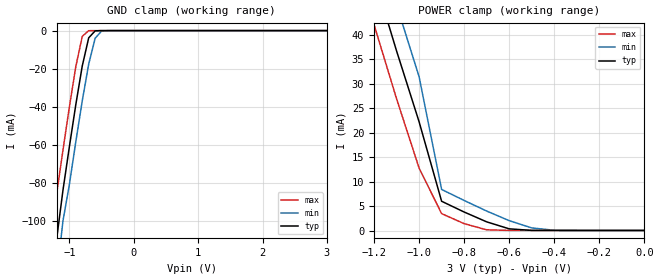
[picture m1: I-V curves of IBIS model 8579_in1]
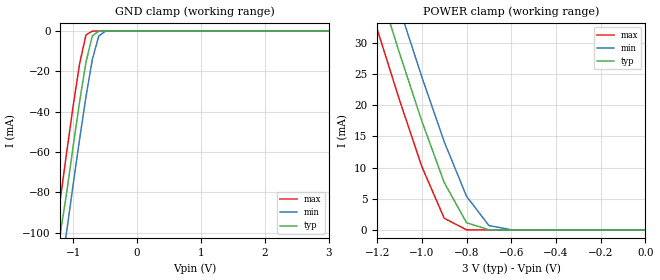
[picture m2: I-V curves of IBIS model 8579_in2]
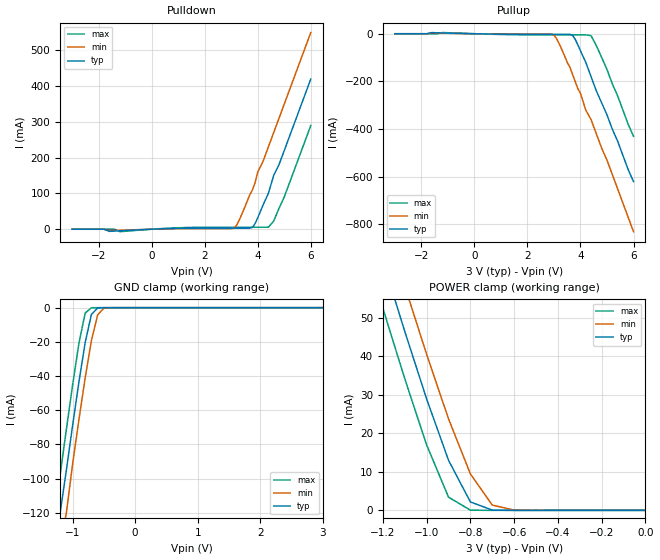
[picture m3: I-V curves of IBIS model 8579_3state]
| IBIS file 4574_3.ibs
[IBIS ver]   3.0
[File name]   4574_3.ibs
[File Rev]   3.0
[Date]   Thursday 7, 2005
[Source]   Hspice simulation by NPC using HA8579 schematics
[Disclaimer]   Data is for modeling purpose only and is not guaranteed.
[Copyright]   SEIKO EPSON Corp.
|   Component RTC-4574SA
[Component]   RTC-4574SA
[Manufacturer]   Seiko Epson Corporation
[Package]
| variable   typ   min   max
R_pkg   3.00m   NA   NA
L_pkg   3.70nH   NA   NA
C_pkg   0.70pF   NA   NA
[Pin]  signal_name   model_name   R_pin   L_pin   C_pin
1   VSS   GND
2   FOUT   8579_3state
|3   NC
|4   NC
|5   NC
|6   NC
7   VDD   POWER
8   CE0   8579_in1
9   AIRQN   8579_od
10   TIRQN   8579_od
11   CLK   8579_in2
12   DATA   8579_io
13   CE1   8579_in2
14   FCON   8579_in2
| Models and submodels in the file (5): 8579_in1 (Input), 8579_in2 (Input), 8579_3state (3-state), 8579_io (I/O), 8579_od (Open_drain)
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|   Model 8579_in1
[Model]   8579_in1
Model_type   Input
Vinl =   0.60V
Vinh =   2.40V
C_comp   8.00pF   8.00pF   8.00pF
[Temperature Range]   25.00   85.00   -40.00
[Voltage Range]   3.00V   2.70V   3.30V
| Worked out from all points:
|   GND clamp passes 1 mA (typ) near -0.62 V on its own axis
|   POWER clamp passes 1 mA (typ) near -0.65 V on its own axis
[GND_clamp]
| voltage   I(typ)   I(min)   I(max)
-3V       -550mA     -570mA     -530mA
-1.3V     -130mA     -150mA     -110mA
-1.2V     -110mA     -130mA     -86.2mA
-1.1V     -83.87mA   -100mA     -62.79mA
-1V       -60.92mA   -80.78mA   -40.05mA
-900mV    -38.82mA   -58.3mA    -18.83mA
-800mV    -18.56mA   -36.84mA   -3.02mA
-700mV    -3.78mA    -17.56mA   -37.75uA
-600mV    -140uA     -3.99mA    -260nA
-500mV    -2.83uA    -250uA     -1.81nA
3V        8.96uA     6.98uA     16.13uA
[POWER_clamp]
| voltage   I(typ)   I(min)   I(max)
-3V       340mA      350mA      340mA
-1.2V     51.94mA    61.35mA    42.1mA
-1.1V     36.73mA    46.14mA    26.95mA
-1V       22.24mA    31.45mA    12.77mA
-900mV    5.98mA     8.4mA      3.45mA
-800mV    3.78mA     6.14mA     1.4mA
-700mV    1.77mA     3.98mA     140uA
-600mV    340uA      2.01mA     17.19uA
-500mV    20.1uA     530uA      16.15uA
-400mV    9.2uA      44.36uA    16.14uA
0V        8.96uA     5.37uA     16.13uA
|   Model 8579_in2
[Model]   8579_in2
Model_type   Input
Vinl =   0.60V
Vinh =   2.40V
C_comp   8.00pF   8.00pF   8.00pF
[Temperature Range]   25.00   85.00   -40.00
[Voltage Range]   3.00V   2.70V   3.30V
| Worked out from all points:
|   GND clamp passes 1 mA (typ) near -0.64 V on its own axis
|   POWER clamp passes 1 mA (typ) near -0.79 V on its own axis
[GND_clamp]
| voltage   I(typ)   I(min)   I(max)
-3V       -540mA     -560mA     -520mA
-1.3V     -130mA     -150mA     -110mA
-1.2V     -100mA     -120mA     -82.91mA
-1.1V     -79.74mA   -98.87mA   -59.57mA
-1V       -56.91mA   -75.91mA   -36.97mA
-900mV    -35.02mA   -53.6mA    -16.13mA
-800mV    -15.33mA   -32.47mA   -1.89mA
-700mV    -2.36mA    -13.97mA   -18.95uA
-600mV    -68.66uA   -2.44mA    -130nA
-500mV    -1.41uA    -130uA     -910pA
3V        3pA        2.02nA     2.7pA
[POWER_clamp]
| voltage   I(typ)   I(min)   I(max)
-3V       260mA      270mA      250mA
-1.2V     39.81mA    47.03mA    32.25mA
-1.1V     28.38mA    35.6mA     20.85mA
-1V       17.46mA    24.55mA    10.16mA
-900mV    7.61mA     14.16mA    1.88mA
-800mV    1.16mA     5.39mA     27.3uA
-700mV    33.67uA    710uA      190nA
-600mV    690nA      33.17uA    1.31nA
0V        3pA        14.76pA    3.3pA
|   Model   8579_3state
[Model]   8579_3state
Model_type   3-state
Polarity   Inverting
C_comp   8.00pF   8.00pF   8.00pF
[Temperature Range]   25   85   -40
[Voltage Range]   3.00V   2.70V   3.30V
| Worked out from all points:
|   slope of the pulldown table from 0 to 0.45 V, typ, clamps not added: 346 ohm
|   slope of the pullup table from 0 to 0.45 V, typ, clamps not added: 474 ohm
|   GND clamp passes 1 mA (typ) near -0.62 V on its own axis
|   POWER clamp passes 1 mA (typ) near -0.74 V on its own axis
[Pulldown]
|   voltage   I(typ)   I(min)   I(max)
-3V       0A         0A         0A
-1.4V     -5.09mA    -3.39mA    0A
-1.2V     -4.49mA    -2.98mA    -6.79mA
3.1V      2.89mA     2.77mA     5.47mA
3.3V      2.9mA      25.15mA    5.48mA
3.8V      5.09mA     110mA      5.49mA
3.9V      15.91mA    130mA      5.49mA
4V        31.8mA     160mA      5.49mA
4.4V      100mA      230mA      5.55mA
4.6V      150mA      270mA      22.48mA
5V        220mA      350mA      90.27mA
6V        420mA      550mA      290mA
[Pullup]
|   voltage   I(typ)   I(min)   I(max)
-3V       0A         0A         0A
-1.2V     3.25mA     2.18mA     5.03mA
3V        -2.47mA    -5.37mA    -4.82mA
3.2V      -2.48mA    -42.34mA   -4.84mA
3.7V      -6.45mA    -170mA     -4.87mA
3.9V      -46.01mA   -230mA     -4.88mA
4V        -71.24mA   -250mA     -4.89mA
4.2V      -120mA     -320mA     -4.9mA
4.4V      -180mA     -360mA     -8.08mA
4.6V      -240mA     -420mA     -50mA
5V        -340mA     -530mA     -150mA
6V        -620mA     -830mA     -430mA
[GND_clamp]
|   voltage   I(typ)   I(min)   I(max)
-3V       -620mA     -650mA     -600mA
-1.3V     -150mA     -170mA     -120mA
-1.2V     -120mA     -140mA     -97.79mA
-1.1V     -94.94mA   -120mA     -71.05mA
-1V       -68.74mA   -91.25mA   -45.09mA
-900mV    -43.52mA   -65.59mA   -20.92mA
-800mV    -20.48mA   -41.13mA   -3.17mA
-700mV    -3.96mA    -19.25mA   -37.79uA
-600mV    -140uA     -4.17mA    -260nA
-500mV    -2.83uA    -250uA     -1.81nA
3V        3.01pA     66.2uA     2.4pA
[POWER_clamp]
|   voltage   I(typ)   I(min)   I(max)
-3V       420mA      430mA      400mA
-1.3V     83.45mA    95.19mA    71.21mA
-1.2V     64.75mA    76.53mA    52.43mA
-1.1V     46.44mA    58.21mA    34.17mA
-1V       28.9mA     40.47mA    16.98mA
-900mV    13mA       23.75mA    3.42mA
-800mV    2.18mA     9.45mA     54.44uA
-700mV    67.16uA    1.37mA     380nA
-600mV    1.39uA     66.2uA     2.63nA
0V        3.01pA     26.51pA    3.6pA
[Ramp]
|variable   typ   min   max
dV/dt_r   1.65/1.36n   1.25/2.23n   2.05/0.80n
dV/dt_f   1.69/1.36n   1.30/2.22n   2.08/0.92n
R_load = 5.00k
| End [Model] 8579_3state
